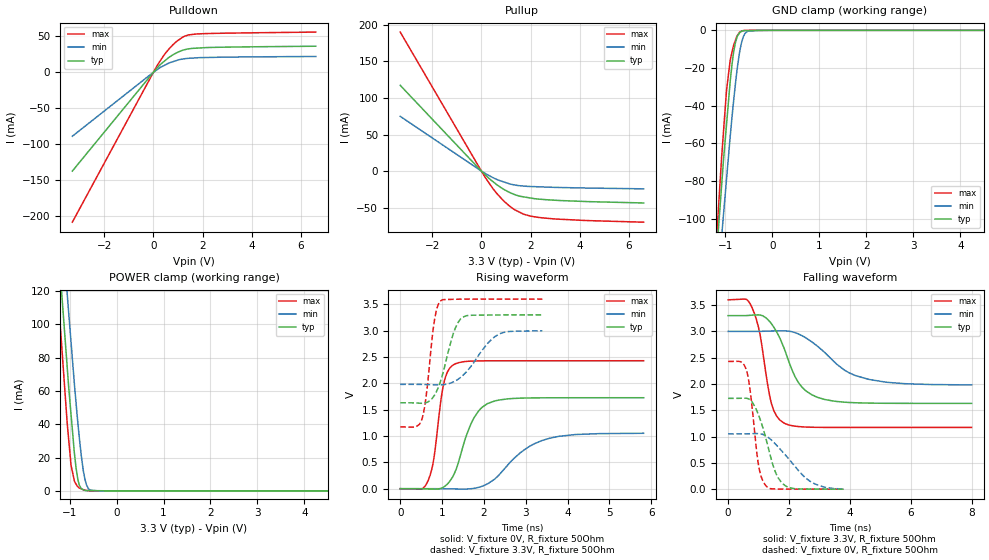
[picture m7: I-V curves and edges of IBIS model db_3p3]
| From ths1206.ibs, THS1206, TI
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|   db_3p3 Model
[Model]   db_3p3
Model_type   I/O
Polarity   Non-Inverting
Enable   Active-High
Vinl = 0.6
Vinh = 2
Vmeas = 1.65
Vref = 1.65
Cref = 30pF
Rref = 50
|   typ   min   max
|   (nom PVT)   (fast PVT)   (slow PVT)
C_comp   1.862e-12   1.857e-12   1.910e-12
|ON state : BUFFER OUTPUT TURNED HIGH
|C_comp   1.967e-12   1.967e-12   2.046e-12
|OFF state: BUFFER IN HIGH IMPEDANCE
|C_comp   1.756e-12   1.747e-12   1.775e-12
| Where nom  PVT is Nominal Process, 3.3V, 43C
|   Fast PVT is Strong Process,  3.6V, -55C
|   Slow PVT is Weak Process,   3V, 145C
[Voltage Range]   3.3   3   3.6
|Ambient Temperature   25   125   -55
|Junction Temperature
[Temperature Range]   43   145   -55
[Pullup Reference]   3.3   3   3.6
[Pulldown Reference]   0   0   0
[Power Clamp Reference]   3.3   3   3.6
[GND Clamp Reference]   0   0   0
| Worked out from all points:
|   slope of the pulldown table from 0 to 0.495 V, typ, clamps not added: 29.4 ohm
|   slope of the pullup table from 0 to 0.495 V, typ, clamps not added: 32.9 ohm
|   GND clamp passes 1 mA (typ) near -0.68 V on its own axis
|   POWER clamp passes 1 mA (typ) near -0.73 V on its own axis
|   falling waveform, V_fixture 3.3V, R_fixture 50Ohm: 20-80 % time 776ps typ, 1.32ns min, 430ps max; typ from 3.3 V to 1.63 V
|   rising waveform, V_fixture 0V, R_fixture 50Ohm: 20-80 % time 469ps typ, 882ps min, 243ps max; typ from 0 V to 1.73 V
|   rising waveform, V_fixture 3.3V, R_fixture 50Ohm: 20-80 % time 348ps typ, 594ps min, 200ps max; typ from 1.63 V to 3.3 V
|   falling waveform, V_fixture 0V, R_fixture 50Ohm: 20-80 % time 523ps typ, 967ps min, 284ps max; typ from 1.73 V to 0 V
[Pulldown]
|   Voltage   I(typ)   I(min)   I(max)
-3.3V     -137.7mA   -89.15mA   -208.8mA
154.8mV   6.085mA    3.721mA    9.471mA
478.8mV   16.39mA    10.14mA    26.04mA
633.6mV   20.75mA    12.87mA    32.52mA
939.6mV   27.02mA    16.33mA    42.83mA
1.246V    31.14mA    18.66mA    49.83mA
1.706V    33.42mA    19.94mA    53.1mA
6.6V      36.19mA    21.93mA    55.87mA
[GND Clamp]
|   Voltage   I(typ)   I(min)   I(max)
-3.3V     -983.3mA   -935.5mA   -1.082A
-1.238V   -136mA     -160.1mA   -130.9mA
-1.084V   -83.6mA    -110.9mA   -68.83mA
-1.065V   -77.27mA   -105.2mA   -62.37mA
-975.6mV  -50mA      -79.1mA    -31.92mA
-896.4mV  -26.84mA   -56.03mA   -15.68mA
-831.6mV  -12.84mA   -39.18mA   -8.589mA
-785.4mV  -6.426mA   -28.19mA   -5.214mA
-694.8mV  -1.23mA    -11.23mA   -879.1uA
-576mV    -201.8uA   -1.477mA   -21.86uA
-285mV    -99.28uA   -1.186uA   -40.77nA
6.6V      0A         0A         0A
[Pullup]
|   Voltage   I(typ)   I(min)   I(max)
-3.3V     117.3mA    74.86mA    190.1mA
172.8mV   -5.77mA    -3.558mA   -9.533mA
633.6mV   -18.81mA   -11.56mA   -30.88mA
903.6mV   -24.8mA    -14.77mA   -40.72mA
1.17V     -29.54mA   -17.74mA   -48.56mA
1.357V    -32.2mA    -19.09mA   -52.98mA
1.706V    -35.22mA   -20.46mA   -58.84mA
2.473V    -38.74mA   -21.71mA   -63.99mA
4.162V    -41.55mA   -23.13mA   -67.49mA
6.6V      -43.63mA   -24.31mA   -69.93mA
[POWER Clamp]
|   Voltage   I(typ)   I(min)   I(max)
-3.3V     1.051A     1.06A      1.062A
-1.426V   222.8mA    265.1mA    197mA
-1.233V   144.7mA    187.8mA    114.3mA
-1.198V   130.5mA    174.5mA    99.32mA
-1.048V   73.41mA    117.5mA    39.91mA
-968.4mV  46.03mA    89.41mA    15.51mA
-897.6mV  22.87mA    64.44mA    5.995mA
-825mV    7.177mA    41.44mA    2.609mA
-691.2mV  549.2uA    9.744mA    522uA
-591mV    198.7uA    1.199mA    100.1uA
-369mV    123.6uA    3.307uA    245.4nA
6.6V      0A         0A         0A
[Ramp]
R_load = 50
|   typ   min   max
dV/dt_r   1.036/4.6594e-10   0.631149/8.79824e-10   1.45735/2.41303e-10
dV/dt_f   1.00125/7.70515e-10   0.610521/1.31284e-09   1.45578/4.28385e-10
[Falling Waveform]
V_fixture = 3.3V
V_fixture_min = 3V
V_fixture_max = 3.6V
R_fixture = 50Ohm
|   Time   V(typ)   V(min)   V(max)
0s        3.3V       3V         3.6V
586ps     3.301V     3V         3.611V
780ps     3.309V     3V         3.459V
1.046ns   3.311V     3.001V     2.946V
1.43ns    3.139V     3.008V     1.614V
1.838ns   2.681V     3.01V      1.257V
2.428ns   1.938V     2.918V     1.185V
3.162ns   1.707V     2.605V     1.175V
4.632ns   1.636V     2.086V     1.174V
7.998ns   1.631V     1.982V     1.174V
[Rising Waveform]
V_fixture = 0V
V_fixture_min = 0V
V_fixture_max = 0V
R_fixture = 50Ohm
|   Time   V(typ)   V(min)   V(max)
0s        1.497nV    4.504nV    1.191nV
504ps     -628uV     174.8uV    -8.094mV
668ps     -4.407mV   237.8uV    156.1mV
810ps     -8.75mV    41.88uV    605.1mV
1.05ns    37.9mV     -1.547mV   2.029V
1.292ns   285.7mV    -4.485mV   2.361V
1.736ns   1.306V     3.044mV    2.423V
2.1ns     1.62V      97.81mV    2.428V
3.384ns   1.725V     913.1mV    2.429V
5.818ns   1.727V     1.052V     2.429V
[Rising Waveform]
V_fixture = 3.3V
V_fixture_min = 3V
V_fixture_max = 3.6V
R_fixture = 50Ohm
|   Time   V(typ)   V(min)   V(max)
0s        1.631V     1.981V     1.174V
376ps     1.627V     1.981V     1.176V
518ps     1.622V     1.979V     1.32V
624ps     1.635V     1.977V     1.788V
796ps     1.747V     1.972V     3.083V
948ps     2.005V     1.971V     3.553V
1.264ns   2.935V     2.024V     3.595V
1.494ns   3.257V     2.148V     3.598V
2.342ns   3.298V     2.927V     3.6V
3.398ns   3.3V       2.998V     3.6V
[Falling Waveform]
V_fixture = 0V
V_fixture_min = 0V
V_fixture_max = 0V
R_fixture = 50Ohm
|   Time   V(typ)   V(min)   V(max)
0s        1.727V     1.052V     2.429V
428ps     1.729V     1.052V     2.42V
612ps     1.728V     1.053V     2.241V
736ps     1.69V      1.055V     1.816V
982ps     1.435V     1.057V     515.9mV
1.234ns   977.6mV    1.016V     69.23mV
1.568ns   303.1mV    848.7mV    3.852mV
1.882ns   62.58mV    649.1mV    1.341mV
2.678ns   2.4mV      155.1mV    208.6uV
3.786ns   332.1uV    3.502mV    130.4uV
